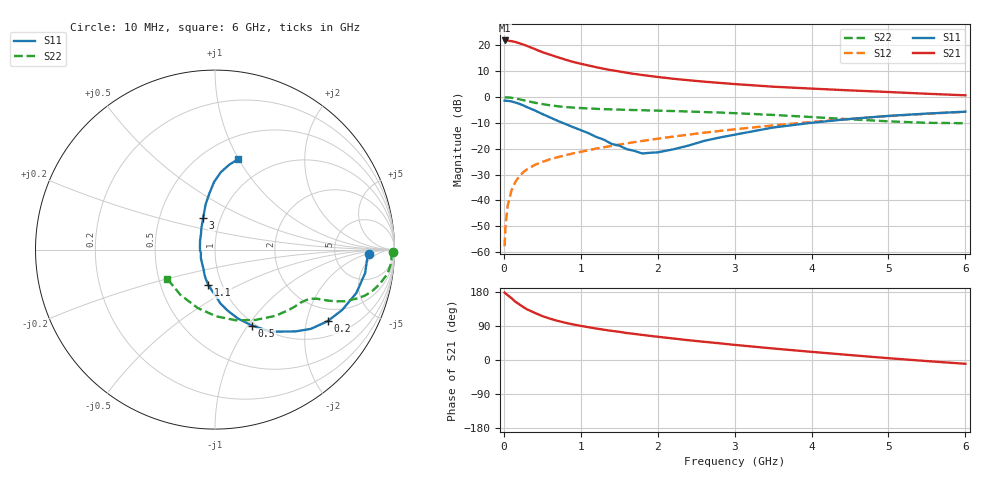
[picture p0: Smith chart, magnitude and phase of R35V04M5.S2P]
! SIEMENS Small Signal Semiconductors
! BFR181
! Si NPN RF Bipolar Junction Transistor in SOT23
! VCE = 5 V  IC = 4.5 mA
! Common Emitter S-Parameters:  May  1996
# GHz  S  MA  R  50
!  f  S11  S21  S12  S22
! GHz  MAG  ANG  MAG  ANG  MAG  ANG  MAG  ANG
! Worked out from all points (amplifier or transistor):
!   36 points, 10 MHz to 6 GHz, reference 50 ohm
!   highest |S21| = 21.9 dB at 10 MHz (marker M1)
!   |S21| within 3 dB of that: start of sweep to 374.8 MHz
!   unconditionally stable (mu >= 1): 1.22 GHz to 3.052 GHz
!   at 250 MHz: K = 0.38, MSG = 24.8 dB, |S12| = -29.1 dB
!   at 1.4 GHz: K = 1.03, MAG = 13.5 dB, |S12| = -18.9 dB
!   at 6 GHz: K = 0.86, MSG = 3.2 dB, |S12| = -5.7 dB
!   S11 on the Smith chart (normalised r, x): 10 MHz: 13, -2; 200 MHz: 1.50, -2.67; 500 MHz: 0.96, -1.04; 1.1 GHz: 0.86, -0.35; 3 GHz: 0.83, +0.30; 6 GHz: 0.72, +1.00
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0.01  0.8577 -1.7  12.48 178.0  0.0013 90.1  0.9919 -0.8
0.02  0.8494 -3.5  12.47 176.1  0.003 88.7  0.9828 -1.7
0.05  0.8466 -8.9  12.37 171.1  0.008 84.7  0.9859 -4.1
0.1  0.8238 -17.1  12.09 163.0  0.0157 80.6  0.9702 -8.0
0.15  0.7847 -25.3  11.66 153.9  0.0228 75.4  0.9388 -11.7
0.2  0.7432 -32.5  11.03 147.1  0.0291 73.3  0.9079 -14.6
0.25  0.6928 -39.6  10.45 140.0  0.0349 70.6  0.8746 -17.0
0.3  0.6401 -45.4  9.795 133.9  0.0399 68.4  0.8392 -18.9
0.4  0.5537 -55.7  8.533 124.6  0.0484 65.0  0.7788 -21.7
0.5  0.4703 -64.1  7.411 115.9  0.0555 63.5  0.732 -23.2
0.6  0.404 -71.7  6.617 109.0  0.0627 62.7  0.6945 -24.2
0.7  0.347 -78.3  5.915 103.3  0.0686 62.5  0.6641 -24.9
0.8  0.3017 -84.3  5.306 98.2  0.0748 62.3  0.6424 -25.4
0.9  0.262 -88.6  4.798 93.9  0.0812 62.3  0.6259 -25.9
1.1  0.2006 -100.6  4.09 86.5  0.0937 63.0  0.6022 -27.1
1.6  0.0979 -140.5  2.95 71.1  0.1273 63.2  0.5662 -31.0
2.2  0.0972 149.0  2.264 56.8  0.1718 62.0  0.5363 -37.9
3  0.1869 110.8  1.787 39.9  0.2378 57.7  0.4882 -50.0
3.5  0.2576 101.7  1.59 30.4  0.2825 53.9  0.4514 -60.3
4.5  0.3779 90.7  1.347 13.0  0.3794 44.0  0.3717 -89.0
5.5  0.4792 80.5  1.16 -2.9  0.4755 31.5  0.3175 -127.1
6  0.5218 75.5  1.082 -10.0  0.5197 24.6  0.312 -148.2
